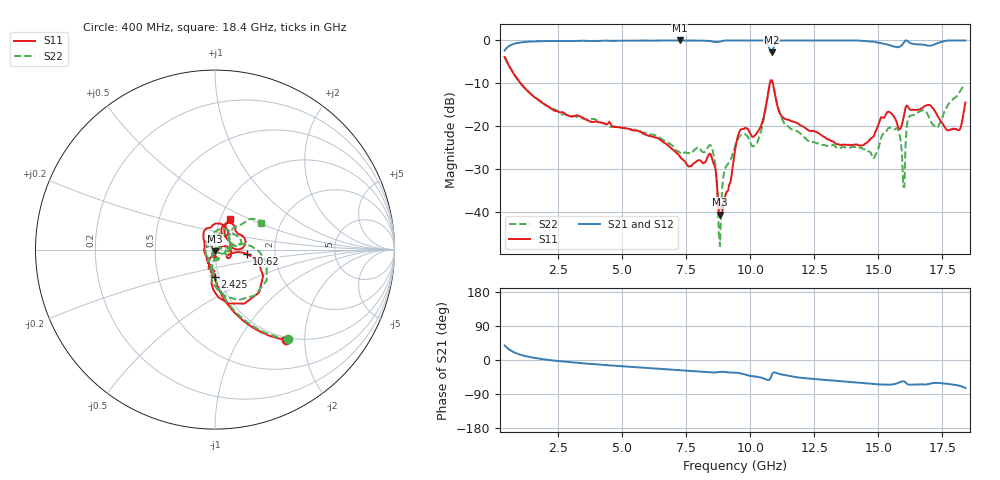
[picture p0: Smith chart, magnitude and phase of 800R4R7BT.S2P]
!  American Technical Ceramics  Date:  10/25/10
!  One Norden Lane
!  Huntington Station,  NY.  11746-2102
!  Tel:  (631) 622-4700  Fax:  (631) 622-4748
!  Part Number  800R4R7BT  Mounting Orientation: Vertical
!  Description: Ultra Low ESR Microwave Capacitor
!  Application: Coupling, Bypass, Tuning, DC Block, Filters, Matching
# GHZ S DB R 50
! Freq  |S11|  S11 Ph  |S21|  S21 Ph  |S12|  S12 Ph  |S22|  S22 Ph
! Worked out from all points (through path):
!   401 points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, 400 MHz to 18.4 GHz, reference 50 ohm
!   highest |S21| = 0.00 dB at 7.24 GHz (marker M1); lowest = -2.8 dB at 10.84 GHz (marker M2)
!   group delay of S21, straight-line fit = 12.9 ps
!   lowest |S11| = -40.6 dB at 8.815 GHz (marker M3), VSWR 1.02, Z = 50.2 - j0.918 ohm
!   |S11| at or under -10 dB: 1.023 GHz to 10.76 GHz (9.74 GHz wide, 165 % of centre); 10.88 GHz to end of sweep
!   |S22| runs from -48.0 to -3.8 dB; largest |S21 - S12| = 0.007
!   S11 on the Smith chart (normalised r, x): 400 MHz: 0.95, -1.63; 2.425 GHz: 0.96, -0.29; 10.62 GHz: 1.42, -0.07; 18.4 GHz: 1.11, +0.39
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0.4  -3.87 -51.9  -2.36 38.2  -2.40 38.2  -3.81 -50.9
2.425  -16.46 -90.1  -0.14 -2.2  -0.17 -2.1  -16.34 -91.9
3.415  -17.90 -99.9  -0.07 -8.4  -0.10 -8.3  -18.15 -96.3
6.43  -22.96 -117.8  -0.02 -23.0  -0.02 -22.8  -22.57 -98.8
7.24  -27.02 -116.4  0.00 -26.9  -0.01 -26.7  -26.15 -86.0
8.455  -26.62 -96.4  -0.19 -32.8  -0.16 -32.6  -24.49 -83.8
8.815  -40.64 -80.2  -0.27 -31.3  -0.25 -31.1  -48.03 79.7
8.995  -36.72 -21.3  -0.01 -31.5  -0.01 -31.3  -30.20 17.8
9.4  -25.70 22.5  -0.01 -33.5  -0.01 -33.2  -24.66 13.2
10.21  -21.95 -21.0  -0.01 -43.6  -0.01 -43.5  -24.34 -3.6
10.615  -15.03 -7.4  -0.37 -51.1  -0.36 -51.1  -15.50 10.4
10.84  -9.30 -61.3  -2.78 -38.6  -2.76 -38.5  -9.40 -49.0
11.335  -18.26 -91.5  -0.01 -39.4  -0.01 -39.4  -19.48 -99.4
12.415  -21.17 -110.0  -0.01 -49.5  -0.01 -49.6  -23.76 -120.2
14.35  -24.47 166.4  -0.06 -60.5  -0.03 -60.6  -25.07 -160.6
15.43  -16.67 76.0  -1.09 -65.1  -1.07 -65.4  -20.32 57.0
15.79  -20.56 53.8  -1.57 -59.9  -1.54 -60.1  -21.18 5.2
15.97  -18.41 72.6  -0.72 -56.1  -0.69 -56.3  -34.10 -52.7
16.24  -16.19 43.6  -0.59 -65.3  -0.57 -65.5  -17.64 53.3
17.32  -17.66 0.3  -0.61 -60.4  -0.58 -60.6  -20.26 32.8
18.085  -20.87 35.7  -0.01 -66.7  -0.01 -67.0  -12.83 42.4
18.4  -14.50 63.4  -0.01 -73.9  -0.01 -74.2  -10.57 29.9
